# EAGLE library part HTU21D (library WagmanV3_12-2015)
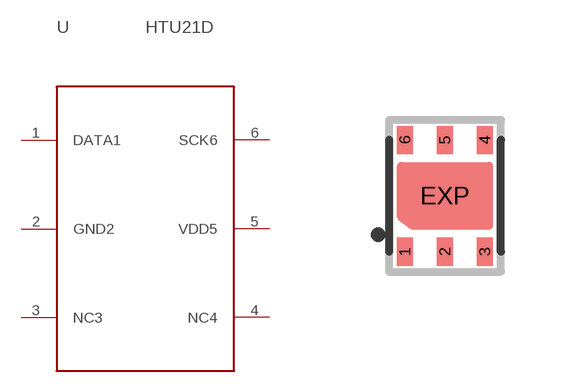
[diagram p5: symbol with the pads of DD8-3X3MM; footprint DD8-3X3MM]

Designator prefix U

## HTU21D  [DD8-3X3MM]
1  DATA1
2  GND2
3  NC3
4  NC4
5  VDD5
6  SCK6

## Footprint DD8-3X3MM (pad centres in mm)
DD Package 8-Lead Plastic DFN (3mm × 3mm) (Reference LTC DWG # 05-08-1698 Rev C) Source: Data sheet
smd 0.4 x 0.7: 1 -1,-1.4; 2 0,-1.4; 3 1,-1.4; 4 1,1.4; 5 0,1.4; 6 -1,1.4
smd 1 x 1: EXP 0,0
